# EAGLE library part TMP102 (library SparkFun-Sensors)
Texas Instruments TMP102 Low-Power Digital Temperature Sensor The TMP102 is a digital sensor (I2C a.k.a. TWI), has a resolution of 0.0625°C, and is accurate up to 0.5°C. This is a very handy sensor that requires a very low-current. Datasheet SparkFun Products SparkFun Digital Temperature Sensor Breakout - TMP102 (SEN-11931)
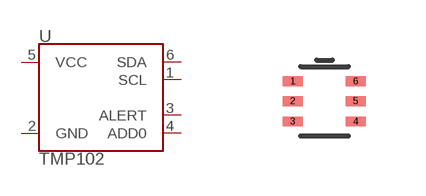
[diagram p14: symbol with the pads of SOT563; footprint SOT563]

Designator prefix U

## TMP102 (PROD_ID: IC-09303)  [SOT563]
1  SCL
2  GND
3  ALERT
4  ADD0
5  VCC
6  SDA

## Footprint SOT563 (pad centres in mm)
6-Pin SOT563 (1:1 Footprint) Datasheet Specifications: Pin Count: 6 Area: 1.7 x 1.7 x 0.5 mm Pitch: 0.5 mm Devices Using: TMP102
smd 0.508 x 0.249: 1 -0.8,0.498; 2 -0.8,0.003; 3 -0.8,-0.506; 4 0.776,-0.506; 5 0.776,0.003; 6 0.776,0.498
